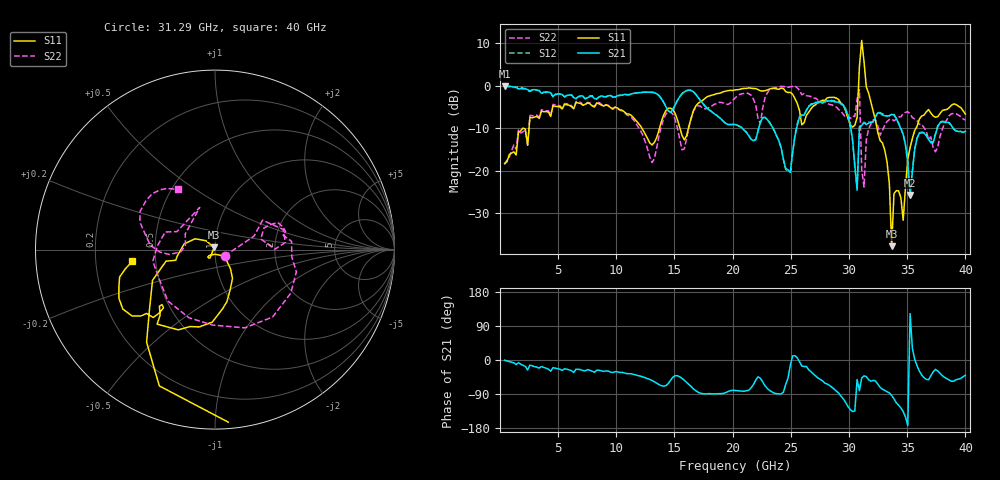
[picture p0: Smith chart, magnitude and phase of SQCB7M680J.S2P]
! Network Analyzer HP8722ES.07.66: Jul 25, 2000 Serial No. US39175408
! 27 Oct 2004  11:18:54
! Frequency  S11  S21  S12  S22
# HZ  S  DB R  50
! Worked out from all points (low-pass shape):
!   201 points, 400 MHz to 40 GHz, reference 50 ohm
!   highest |S21| = -0.08 dB at 400 MHz (marker M1); lowest = -25.7 dB at 35.25 GHz (marker M2)
!   |S21| within 3 dB of the highest: start of sweep to 13.88 GHz; 15.34 GHz to 17.12 GHz (1.782 GHz wide, 11 % of centre)
!   lowest |S11| = -37.8 dB at 33.66 GHz (marker M3), VSWR 1.03, Z = 49.5 + j1.19 ohm
!   |S11| at or under -10 dB: start of sweep to 1.976 GHz; 12.2 GHz to 13.71 GHz (1.517 GHz wide, 11.7 % of centre); 32.4 GHz to 35.76 GHz (3.353 GHz wide, 9.84 % of centre)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
!   |S22| runs from -23.9 to 0.0 dB; largest |S21 - S12| = 0.045
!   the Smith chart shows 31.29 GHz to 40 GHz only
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4e8  -18.30 -94.5  -0.08 -0.6  -0.02 0.3  -18.56 -91.2
7.132e9  -4.60 -108.7  -2.42 -27.9  -2.53 -28.8  -4.48 -122.0
1.3666e10  -10.49 -22.8  -2.31 -64.9  -2.29 -65.2  -11.83 -30.7
2.02e10  -0.98 5.8  -9.10 -80.3  -9.07 -80.5  -2.88 -13.1
2.1784e10  -0.65 -2.0  -12.93 -64.9  -12.91 -65.2  -3.13 -33.9
2.2774e10  -1.16 -3.9  -7.43 -67.8  -7.43 -68.9  -2.87 14.3
2.515e10  -1.99 -64.2  -15.75 10.7  -15.91 7.4  -0.15 -26.5
2.5744e10  -5.83 -130.7  -7.41 -4.2  -7.17 -5.8  -1.04 -25.8
2.6932e10  -4.77 125.8  -4.20 -37.0  -4.14 -39.0  -2.91 -33.9
2.9704e10  -5.87 25.4  -5.46 -111.9  -5.53 -111.9  -7.40 -58.2
3.0694e10  -7.49 51.4  -24.61 -51.6  -23.87 -47.9  -3.12 -133.4
3.0892e10  4.49 34.1  -9.98 -80.9  -9.59 -77.5  -0.92 75.0
3.109e10  10.68 -56.7  -9.33 -47.2  -9.15 -48.7  -19.80 -164.5
3.1288e10  5.70 -84.0  -8.72 -42.0  -8.59 -42.4  -23.86 -33.1
3.1684e10  -1.72 -112.2  -8.79 -52.1  -8.52 -52.7  -10.13 31.7
3.3466e10  -23.11 135.2  -7.05 -86.6  -7.06 -87.9  -7.97 18.4
3.3664e10  -37.80 111.7  -6.74 -93.5  -6.65 -94.8  -7.83 14.3
3.3862e10  -25.42 -120.5  -6.89 -102.5  -6.79 -104.4  -8.26 12.6
3.4654e10  -31.68 -89.3  -11.51 -136.2  -11.41 -136.6  -6.56 -15.3
3.5248e10  -14.54 -58.7  -25.71 122.3  -25.67 119.8  -6.62 -69.2
3.604e10  -7.86 -92.2  -11.22 -28.9  -11.10 -29.3  -9.08 -152.1
4e10  -6.66 -171.8  -10.73 -40.0  -10.68 -39.8  -8.07 121.0
